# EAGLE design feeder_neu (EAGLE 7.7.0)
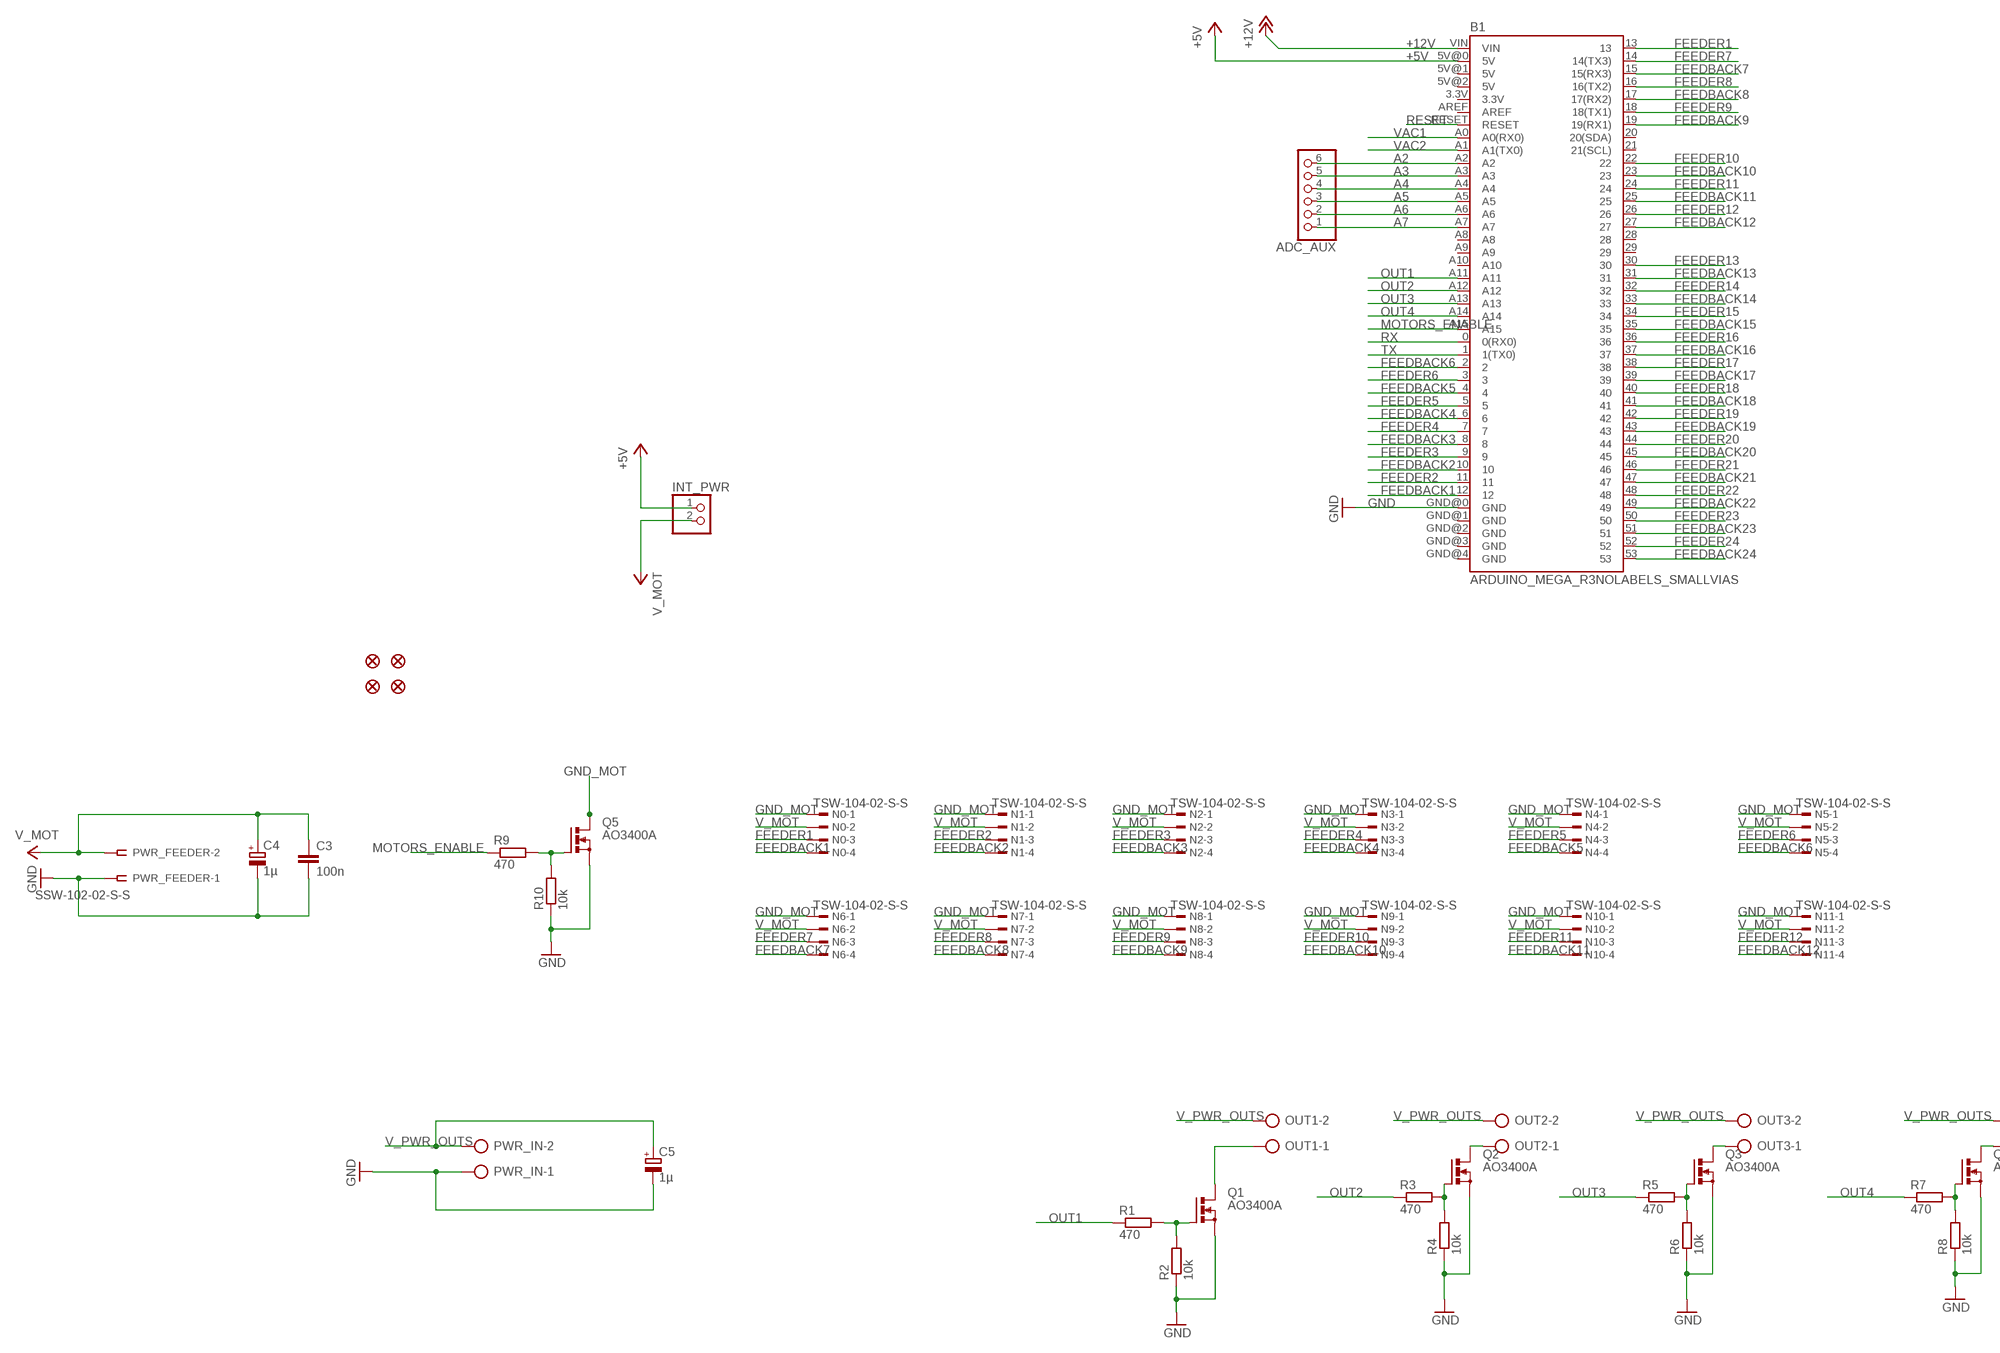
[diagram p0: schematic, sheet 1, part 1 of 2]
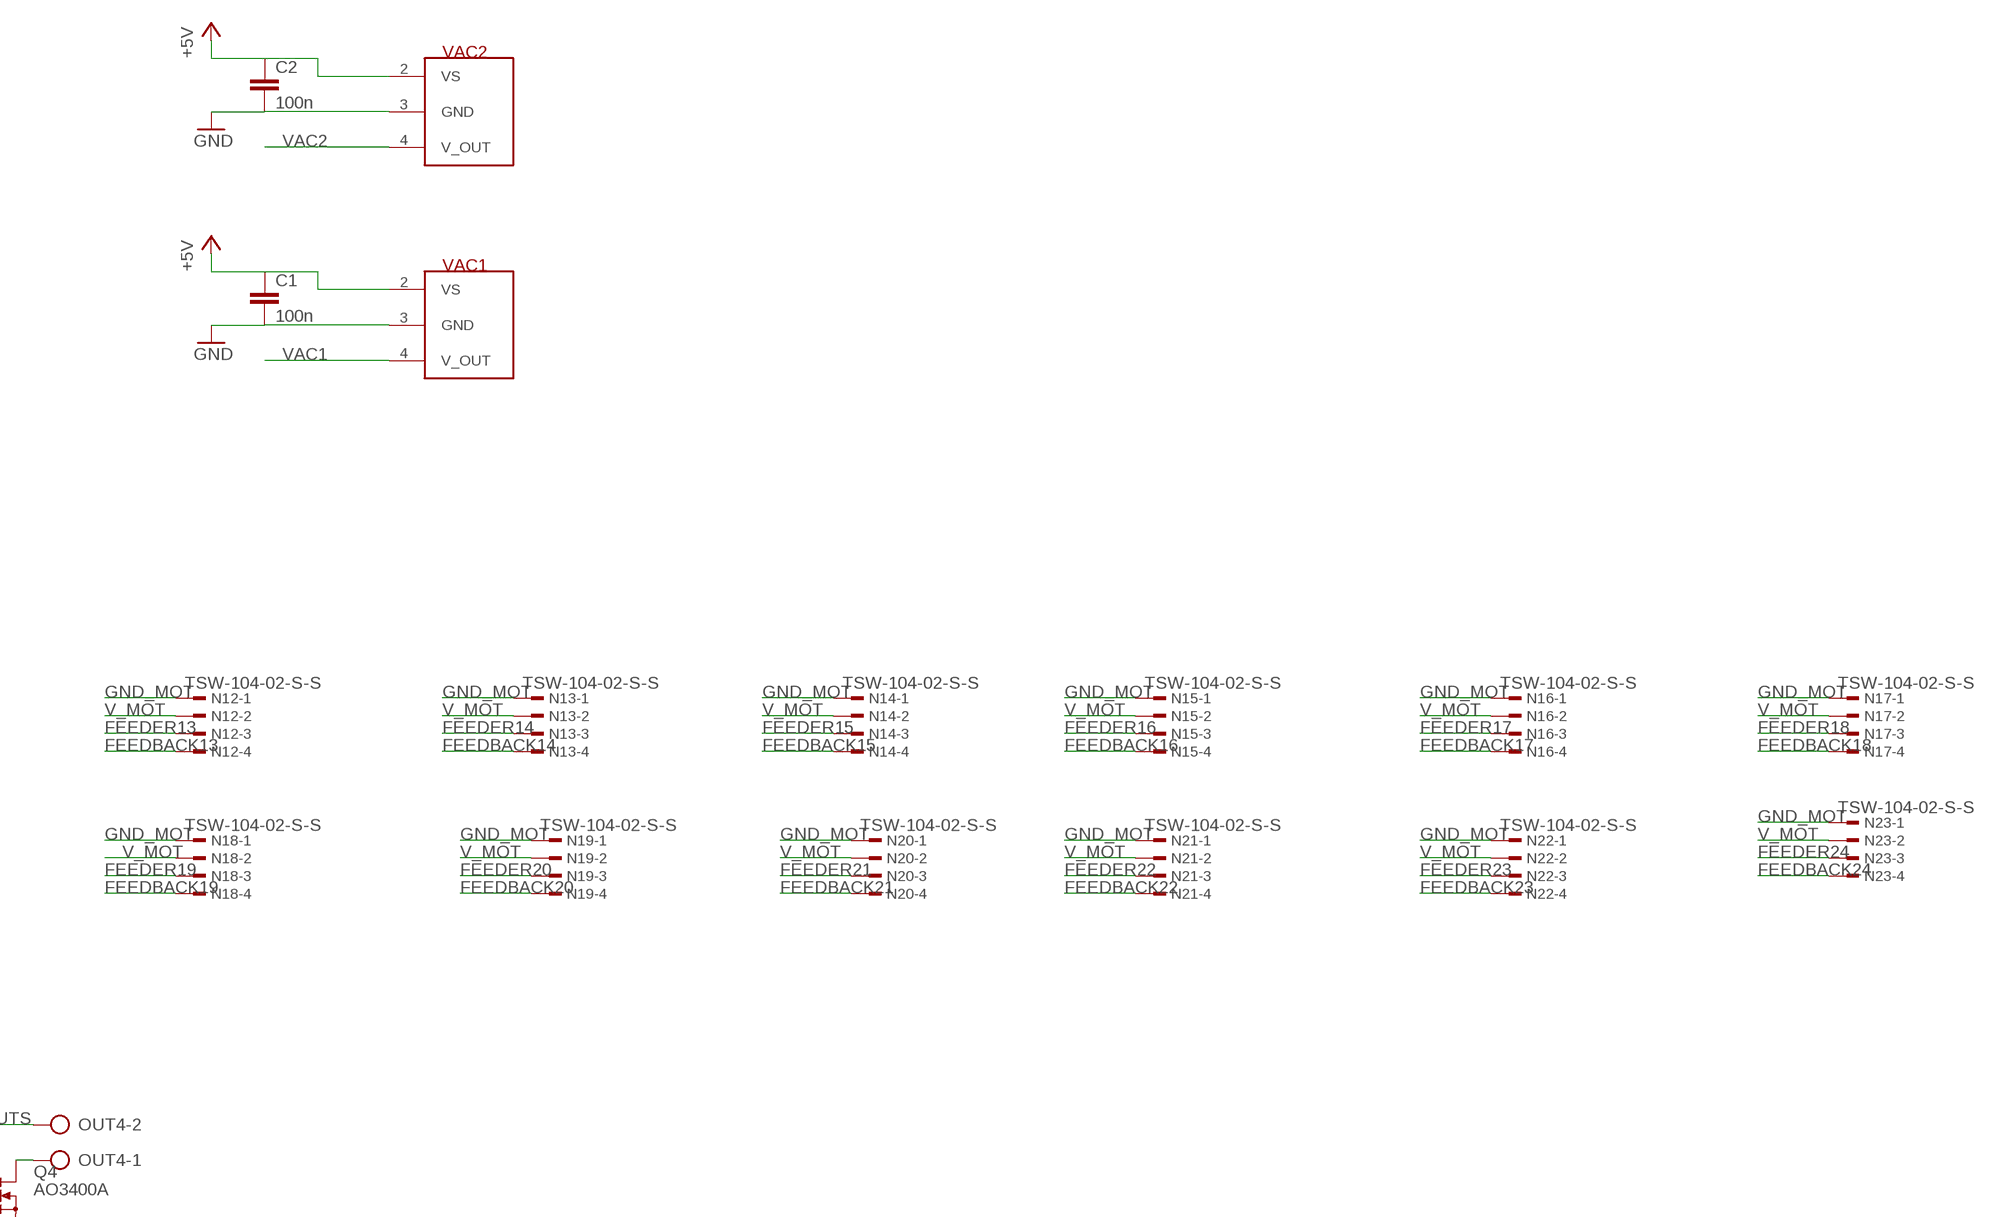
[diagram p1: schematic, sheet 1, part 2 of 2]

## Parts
ADC_AUX  PINHD-1X6  [1X06]
B1  ARDUINO_MEGA_R3NOLABELS_SMALLVIAS  [ARDUINO_MEGA_NOLABELS_SMALLVIAS]
C1  100n  C-EUC0603K  [C0603K]
C2  100n  C-EUC0603K  [C0603K]
C3  100n  C-EUC0603K  [C0603K]
C4  1µ  CPOL-EUE2.5-5  [E2,5-5]
C5  1µ  CPOL-EUE2.5-5  [E2,5-5]
FD1  FIDUCIAL1X2  [FIDUCIAL-1X2]
FD2  FIDUCIAL1X2  [FIDUCIAL-1X2]
FD3  FIDUCIAL1X2  [FIDUCIAL-1X2]
FD4  FIDUCIAL1X2  [FIDUCIAL-1X2]
INT_PWR  PINHD-1X2  [1X02]
N0  TSW-104-02-S-S  [TSW-104-02-S-S]
N1  TSW-104-02-S-S  [TSW-104-02-S-S]
N2  TSW-104-02-S-S  [TSW-104-02-S-S]
N3  TSW-104-02-S-S  [TSW-104-02-S-S]
N4  TSW-104-02-S-S  [TSW-104-02-S-S]
N5  TSW-104-02-S-S  [TSW-104-02-S-S]
N6  TSW-104-02-S-S  [TSW-104-02-S-S]
N7  TSW-104-02-S-S  [TSW-104-02-S-S]
N8  TSW-104-02-S-S  [TSW-104-02-S-S]
N9  TSW-104-02-S-S  [TSW-104-02-S-S]
N10  TSW-104-02-S-S  [TSW-104-02-S-S]
N11  TSW-104-02-S-S  [TSW-104-02-S-S]
N12  TSW-104-02-S-S  [TSW-104-02-S-S]
N13  TSW-104-02-S-S  [TSW-104-02-S-S]
N14  TSW-104-02-S-S  [TSW-104-02-S-S]
N15  TSW-104-02-S-S  [TSW-104-02-S-S]
N16  TSW-104-02-S-S  [TSW-104-02-S-S]
N17  TSW-104-02-S-S  [TSW-104-02-S-S]
N18  TSW-104-02-S-S  [TSW-104-02-S-S]
N19  TSW-104-02-S-S  [TSW-104-02-S-S]
N20  TSW-104-02-S-S  [TSW-104-02-S-S]
N21  TSW-104-02-S-S  [TSW-104-02-S-S]
N22  TSW-104-02-S-S  [TSW-104-02-S-S]
N23  TSW-104-02-S-S  [TSW-104-02-S-S]
OUT1  AK500/2  [AK500/2]
OUT2  AK500/2  [AK500/2]
OUT3  AK500/2  [AK500/2]
OUT4  AK500/2  [AK500/2]
PWR_FEEDER  SSW-102-02-S-S  [SSW-102-02-S-S]
PWR_IN  AK500/2  [AK500/2]
Q1  AO3400A  [SOT23]
Q2  AO3400A  [SOT23]
Q3  AO3400A  [SOT23]
Q4  AO3400A  [SOT23]
Q5  AO3400A  [SOT23]
R1  470  R-EU_R0805  [R0805]
R2  10k  R-EU_R0805  [R0805]
R3  470  R-EU_R0805  [R0805]
R4  10k  R-EU_R0805  [R0805]
R5  470  R-EU_R0805  [R0805]
R6  10k  R-EU_R0805  [R0805]
R7  470  R-EU_R0805  [R0805]
R8  10k  R-EU_R0805  [R0805]
R9  470  R-EU_R0805  [R0805]
R10  10k  R-EU_R0805  [R0805]
VAC1  MPXV6115VC6U  [MPXV6115VC6U]
VAC2  MPXV6115VC6U  [MPXV6115VC6U]

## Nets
+5V: B1.5V@0(5V) C1.1 C2.1 INT_PWR.1 VAC1.2(VS) VAC2.2(VS)
+12V: B1.VIN
A2: ADC_AUX.6 B1.A2
A3: ADC_AUX.5 B1.A3
A4: ADC_AUX.4 B1.A4
A5: ADC_AUX.3 B1.A5
A6: ADC_AUX.2 B1.A6
A7: ADC_AUX.1 B1.A7
FEEDBACK1: B1.12 N0.4
FEEDBACK2: B1.10 N1.4
FEEDBACK3: B1.8 N2.4
FEEDBACK4: B1.6 N3.4
FEEDBACK5: B1.4 N4.4
FEEDBACK6: B1.2 N5.4
FEEDBACK7: B1.15(15(RX3)) N6.4
FEEDBACK8: B1.17(17(RX2)) N7.4
FEEDBACK9: B1.19(19(RX1)) N8.4
FEEDBACK10: B1.23 N9.4
FEEDBACK11: B1.25 N10.4
FEEDBACK12: B1.27 N11.4
FEEDBACK13: B1.31 N12.4
FEEDBACK14: B1.33 N13.4
FEEDBACK15: B1.35 N14.4
FEEDBACK16: B1.37 N15.4
FEEDBACK17: B1.39 N16.4
FEEDBACK18: B1.41 N17.4
FEEDBACK19: B1.43 N18.4
FEEDBACK20: B1.45 N19.4
FEEDBACK21: B1.47 N20.4
FEEDBACK22: B1.49 N21.4
FEEDBACK23: B1.51 N22.4
FEEDBACK24: B1.53 N23.4
FEEDER1: B1.13 N0.3
FEEDER2: B1.11 N1.3
FEEDER3: B1.9 N2.3
FEEDER4: B1.7 N3.3
FEEDER5: B1.5 N4.3
FEEDER6: B1.3 N5.3
FEEDER7: B1.14(14(TX3)) N6.3
FEEDER8: B1.16(16(TX2)) N7.3
FEEDER9: B1.18(18(TX1)) N8.3
FEEDER10: B1.22 N9.3
FEEDER11: B1.24 N10.3
FEEDER12: B1.26 N11.3
FEEDER13: B1.30 N12.3
FEEDER14: B1.32 N13.3
FEEDER15: B1.34 N14.3
FEEDER16: B1.36 N15.3
FEEDER17: B1.38 N16.3
FEEDER18: B1.40 N17.3
FEEDER19: B1.42 N18.3
FEEDER20: B1.44 N19.3
FEEDER21: B1.46 N20.3
FEEDER22: B1.48 N21.3
FEEDER23: B1.50 N22.3
FEEDER24: B1.52 N23.3
GND: B1.GND@0(GND) C1.2 C2.2 C3.2 C4.- C5.- PWR_FEEDER.1 PWR_IN.1 Q1.2(S) Q2.2(S) Q3.2(S) Q4.2(S) Q5.2(S) R2.1 R4.1 R6.1 R8.1 R10.1 VAC1.3(GND) VAC2.3(GND)
GND_MOT: N0.1 N1.1 N2.1 N3.1 N4.1 N5.1 N6.1 N7.1 N8.1 N9.1 N10.1 N11.1 N12.1 N13.1 N14.1 N15.1 N16.1 N17.1 N18.1 N19.1 N20.1 N21.1 N22.1 N23.1 Q5.3(D)
MOTORS_ENABLE: B1.A15 R9.1
N$1: Q1.1(G) R1.2 R2.2
N$2: OUT4.1 Q4.3(D)
N$3: Q5.1(G) R9.2 R10.2
N$4: OUT1.1 Q1.3(D)
N$7: OUT2.1 Q2.3(D)
N$8: OUT3.1 Q3.3(D)
N$10: Q4.1(G) R7.2 R8.2
N$13: Q3.1(G) R5.2 R6.2
N$14: Q2.1(G) R3.2 R4.2
OUT1: B1.A11 R1.1
OUT2: B1.A12 R3.1
OUT3: B1.A13 R5.1
OUT4: B1.A14 R7.1
RESET: B1.RESET
RX: B1.0(0(RX0))
TX: B1.1(1(TX0))
V_MOT: C3.1 C4.+ INT_PWR.2 N0.2 N1.2 N2.2 N3.2 N4.2 N5.2 N6.2 N7.2 N8.2 N9.2 N10.2 N11.2 N12.2 N13.2 N14.2 N15.2 N16.2 N17.2 N18.2 N19.2 N20.2 N21.2 N22.2 N23.2 PWR_FEEDER.2
V_PWR_OUTS: C5.+ OUT1.2 OUT2.2 OUT3.2 OUT4.2 PWR_IN.2
VAC1: B1.A0(A0(RX0)) VAC1.4(V_OUT)
VAC2: B1.A1(A1(TX0)) VAC2.4(V_OUT)
Unconnected: B1.3.3V B1.5V@1(5V) B1.5V@2(5V) B1.20(20(SDA)) B1.21(21(SCL)) B1.28 B1.29 B1.A8 B1.A9 B1.A10 B1.AREF B1.GND@1(GND) B1.GND@2(GND) B1.GND@3(GND) B1.GND@4(GND)

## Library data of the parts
ADC_AUX = pinhead:PINHD-1X6: PIN HEADER
B1 = SparkFun-Boards:ARDUINO_MEGA_R3: Arduino Mega R3 ATmega2560 R3 compatible footprint. SparkFun Products: Arduino Mega 2560 R3
C1-C3 = resistor:C-EU: CAPACITOR, European symbol
C4 C5 = rcl:CPOL-EU: POLARIZED CAPACITOR, European symbol
FD1-FD4 = SparkFun-Aesthetics:FIDUCIAL: Fiducial Alignment Points
INT_PWR = pinhead:PINHD-1X2: PIN HEADER
N0 N1-N23 = con-samtec:TSW-104-02-S-S: THROUGH-HOLE .025" SQ POST HEADER Source: Samtec TSW.pdf; OC_FARNELL: unknown; OC_NEWARK: unknown
OUT1-OUT4 PWR_IN = con-ptr500:AK500/2: CONNECTOR; OC_FARNELL: unknown; OC_NEWARK: unknown
PWR_FEEDER = con-samtec:SSW-102-02-S-S: THROUGH-HOLE .025" SQ POST SOCKET; MPN: SSW-102-02-S-S; OC_FARNELL: unknown; OC_NEWARK: 11P9351
Q1-Q5 = mosfets:AO3400A: N-CHANNEL MOS FET
R1-R10 = resistor:R-EU_: RESISTOR, European symbol
VAC1 VAC2 = sensors:MPXV6115VC6U

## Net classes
0 default: clearance 0.205 mm
2 ledpower: width 0.102 mm, clearance 0.205 mm to class 0, clearance 0.205 mm to class 1, clearance 0.205 mm

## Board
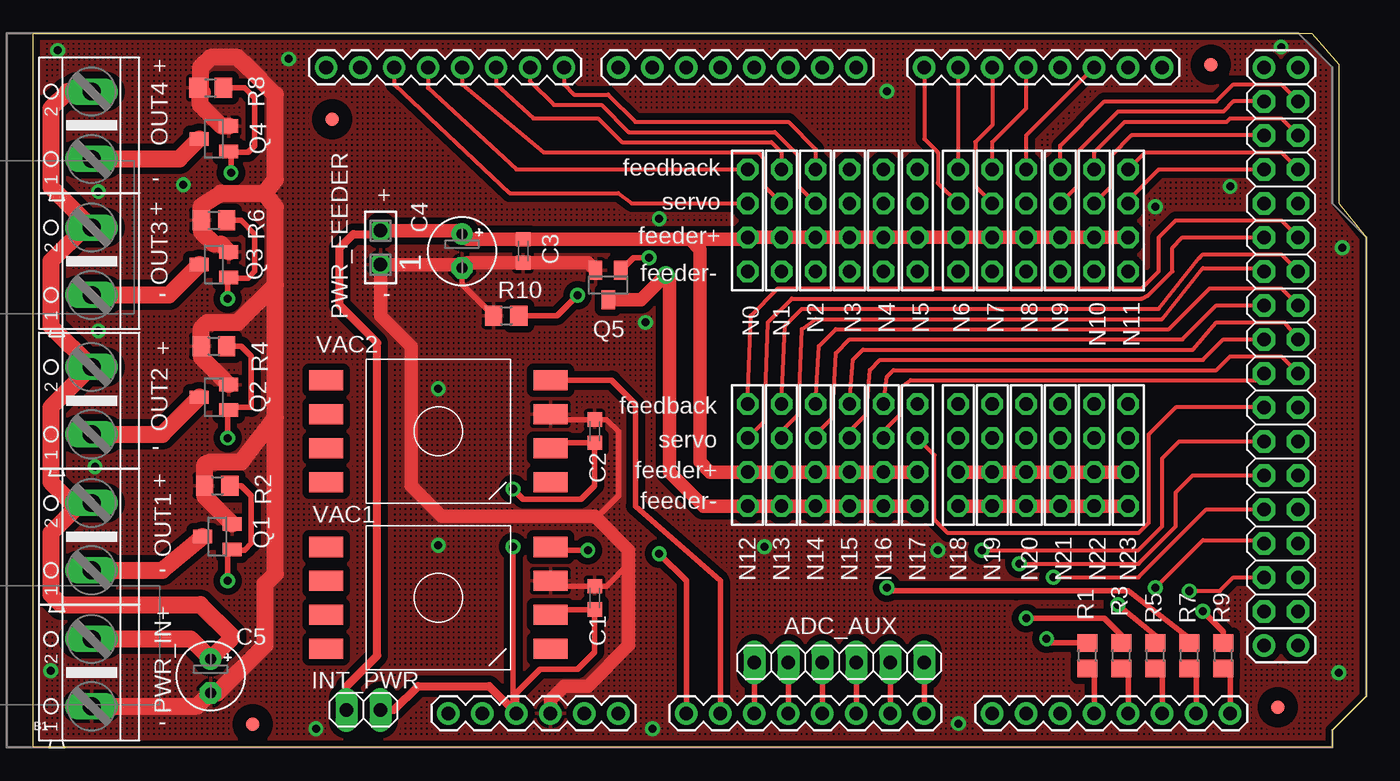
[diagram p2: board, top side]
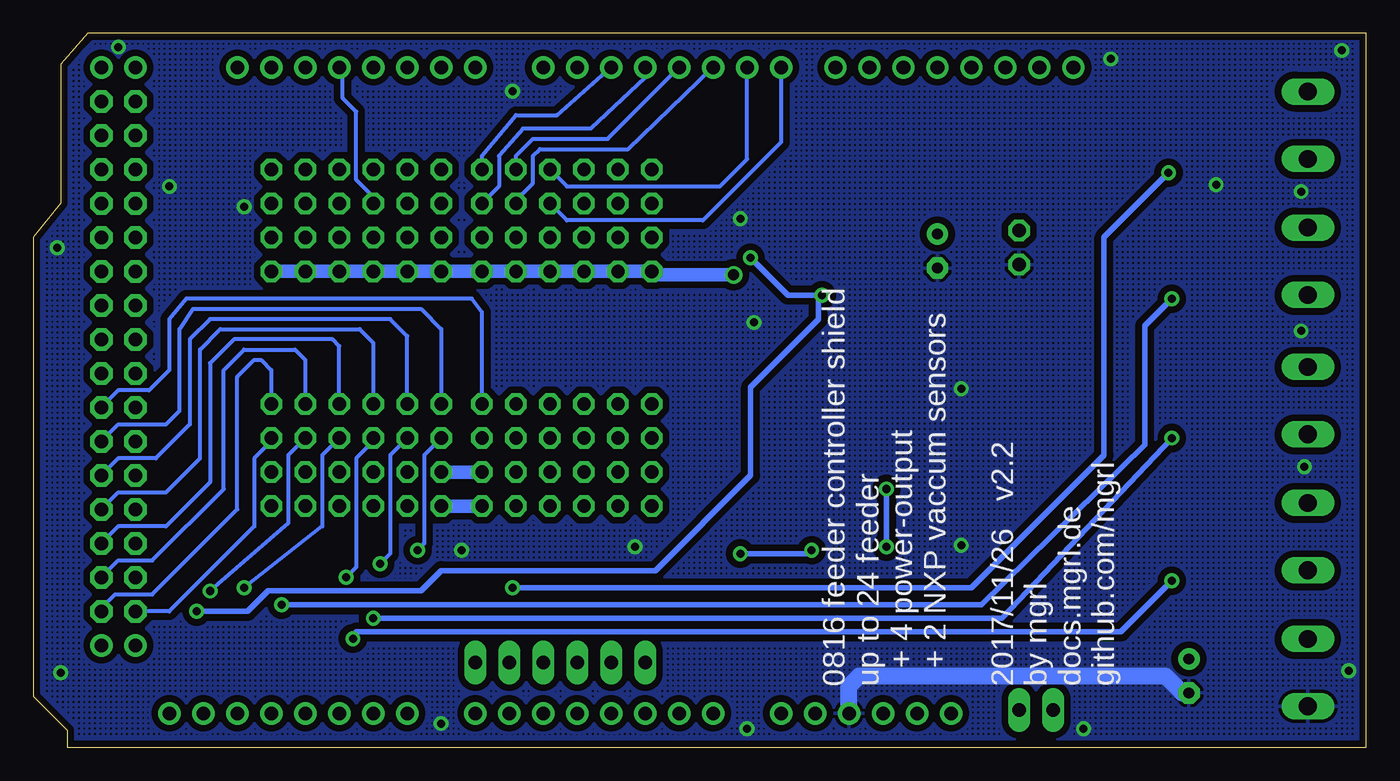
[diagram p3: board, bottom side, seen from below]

Size 99.6 x 53.34 mm. Coordinates in mm from the lower left corner, seen from the top.
Outline: 0,0 0,53.34 95.54,53.34 97.57,51.05 97.57,40.64 99.6,38.1 99.6,3.81 97.06,1.27 97.06,0 0,0
Copper layers (1*16): Top 0.035mm / dielectric 1.5mm / Bottom 0.035mm
Design rules "SparkFun": minimum track width 8mil, minimum drill 20mil, track to track 8mil, track to pad 8mil, pad to pad 8mil, via to via 8mil, smd to smd 8mil, copper to edge 8mil, drill to drill 8mil, minimum pad ring 12mil, minimum via ring 10mil, stop-mask expansion 4mil, vias tented up to drill 20mil, thermal gap 10mil

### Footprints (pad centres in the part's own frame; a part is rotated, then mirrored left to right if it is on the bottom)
1X06 = drill 1.016 long: 1 -6.35,0; 2 -3.81,0; 3 -1.27,0; 4 1.27,0; 5 3.81,0; 6 6.35,0
ARDUINO_MEGA_NOLABELS_SMALLVIAS = drill 1.016 pad 1.676: 0 13.97,24.13; 1 11.43,24.13; 2 8.89,24.13; 3 6.35,24.13; 3.3V -13.97,-24.13; 4 3.81,24.13; 5 1.27,24.13; 5V@0 -11.43,-24.13; 5V@1 44.45,24.13; 5V@2 46.99,24.13; 6 -1.27,24.13; 7 -3.81,24.13; 8 -7.874,24.13; 9 -10.414,24.13; 10 -12.954,24.13; 11 -15.494,24.13; 12 -18.034,24.13; 13 -20.574,24.13; 14 19.05,24.13; 15 21.59,24.13; 16 24.13,24.13; 17 26.67,24.13; 18 29.21,24.13; 19 31.75,24.13; 20 34.29,24.13; 21 36.83,24.13; A0 1.27,-24.13; A1 3.81,-24.13; A2 6.35,-24.13; A3 8.89,-24.13; A4 11.43,-24.13; A5 13.97,-24.13; A6 16.51,-24.13; A7 19.05,-24.13; A8 24.13,-24.13; A9 26.67,-24.13; A10 29.21,-24.13; A11 31.75,-24.13; A12 34.29,-24.13; A13 36.83,-24.13; A14 39.37,-24.13; A15 41.91,-24.13; AREF -25.654,24.13; GND@0 -8.89,-24.13; GND@1 -6.35,-24.13; GND@2 44.45,-19.05; GND@3 46.99,-19.05; GND@4 -23.114,24.13; RESET -16.51,-24.13; VIN -3.81,-24.13 | drill 1.016 pad 1.676 octagon: 22 44.45,21.59; 23 46.99,21.59; 24 44.45,19.05; 25 46.99,19.05; 26 44.45,16.51; 27 46.99,16.51; 28 44.45,13.97; 29 46.99,13.97; 30 44.45,11.43; 31 46.99,11.43; 32 44.45,8.89; 33 46.99,8.89; 34 44.45,6.35; 35 46.99,6.35; 36 44.45,3.81; 37 46.99,3.81; 38 44.45,1.27; 39 46.99,1.27; 40 44.45,-1.27; 41 46.99,-1.27; 42 44.45,-3.81; 43 46.99,-3.81; 44 44.45,-6.35; 45 46.99,-6.35; 46 44.45,-8.89; 47 46.99,-8.89; 48 44.45,-11.43; 49 46.99,-11.43; 50 44.45,-13.97; 51 46.99,-13.97; 52 44.45,-16.51; 53 46.99,-16.51
C0603K = smd 1.05 x 1.08: 1 -0.875,0; 2 0.875,0
E2,5-5 = drill 0.813 pad 1.6: + -1.27,0 | drill 0.813 pad 1.6 octagon: - 1.27,0
FIDUCIAL-1X2 = smd 1 x 1: 1 0,0
1X02 = drill 1.016 long: 1 -1.27,0; 2 1.27,0
TSW-104-02-S-S = drill 1 pad 1.5 octagon: 1 3.81,0; 2 1.27,0; 3 -1.27,0; 4 -3.81,0
AK500/2 = drill 1.321 long: 1 -2.515,0; 2 2.515,0
SSW-102-02-S-S = drill 1 pad 1.5 octagon: 1 -1.27,0; 2 1.27,0
SOT23 = smd 1 x 1.4: 1 -0.95,-1.1; 2 0.95,-1.1; 3 0,1.1
R0805 = smd 1.3 x 1.5: 1 -0.95,0; 2 0.95,0
MPXV6115VC6U = smd 2.54 x 1.524: 1 8.382,-3.81; 2 8.382,-1.27; 3 8.382,1.27; 4 8.382,3.81; 5 -8.382,-3.81; 6 -8.382,-1.27; 7 -8.382,1.27; 8 -8.382,3.81

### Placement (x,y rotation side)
ADC_AUX  60.23,6.35 180 top
B1  47.53,26.67 0 top
C1  41.94,11.18 90 top
C2  41.94,23.62 90 top
C3  36.61,37.08 270 top
C4  32.04,37.08 270 top
C5  13.24,5.33 270 top
FD1  16.38,1.73 0 top
FD2  22.32,46.94 0 top
FD3  93,3 0 top
FD4  88,51 0 top
INT_PWR  24.67,2.79 180 top
N0  53.37,39.37 270 top
N1  55.91,39.37 270 top
N2  58.45,39.37 270 top
N3  60.99,39.37 270 top
N4  63.53,39.37 270 top
N5  66.07,39.37 270 top
N6  69.12,39.37 270 top
N7  71.66,39.37 270 top
N8  74.2,39.37 270 top
N9  76.74,39.37 270 top
N10  79.28,39.37 270 top
N11  81.82,39.37 270 top
N12  53.37,21.84 270 top
N13  55.91,21.84 270 top
N14  58.45,21.84 270 top
N15  60.99,21.84 270 top
N16  63.53,21.84 270 top
N17  66.07,21.84 270 top
N18  69.12,21.84 270 top
N19  71.66,21.84 270 top
N20  74.2,21.84 270 top
N21  76.74,21.84 270 top
N22  79.28,21.84 270 top
N23  81.82,21.84 270 top
OUT1  4.35,15.75 90 top
OUT2  4.35,25.91 90 top
OUT3  4.35,36.32 90 top
OUT4  4.35,46.48 90 top
PWR_FEEDER  25.94,37.34 90 top
PWR_IN  4.35,5.59 90 top
Q1  13.75,15.75 90 top
Q2  13.49,26.16 90 top
Q3  13.49,36.07 90 top
Q4  13.49,45.47 90 top
Q5  42.96,34.54 180 top
R1  78.77,6.86 90 top
R2  13.75,19.56 0 top
R3  81.31,6.86 90 top
R4  13.49,29.97 0 top
R5  83.85,6.86 90 top
R6  13.49,39.37 0 top
R7  86.39,6.86 90 top
R8  13.24,49.28 0 top
R9  88.93,6.86 90 top
R10  35.34,32.26 0 top
VAC1  30.26,11.18 0 top
VAC2  30.26,23.62 0 top

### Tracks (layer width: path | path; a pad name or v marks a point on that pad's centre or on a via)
+5V  (via drill 0.6)
  Top 0.406: VAC1.2 39.03,10.3 C1.1 41.94,7.11 40.67,5.84 37.88,5.84 36.1,4.06 B1.5V@0 35.85,2.79 v35.85,14.99 | v35.85,19.3 36.61,18.54 40.93,18.54 41.94,19.56 C2.1 39.03,22.75 VAC2.2
  Top 0.61: INT_PWR.1 26.96,2.79 28.73,4.57 34.07,4.57 B1.5V@0
  Bottom 0.406: v35.85,19.3 v35.85,14.99
A2
  Top 0.406: B1.A2 ADC_AUX.6
A3
  Top 0.406: B1.A3 ADC_AUX.5
A4
  Top 0.406: B1.A4 ADC_AUX.4
A5
  Top 0.406: B1.A5 ADC_AUX.3
A6
  Top 0.406: B1.A6 ADC_AUX.2
A7
  Top 0.406: B1.A7 ADC_AUX.1
FEEDBACK1
  Top 0.305: B1.12 29.5,49.28 36.1,43.18 37.12,43.18 50.32,43.18 N0.4
FEEDBACK2
  Top 0.305: B1.10 34.58,49.53 37.37,46.99 42.2,46.99 43.97,45.21 55.15,45.21 55.91,44.45 N1.4
FEEDBACK3
  Top 0.305: B1.8 39.66,49.53 40.42,48.77 42.96,48.77 44.99,46.74 56.42,46.74 58.45,44.7 N2.4
FEEDBACK4
  Bottom 0.305: N3.4 59.72,41.91 48.29,41.91 46.26,43.94 B1.6
FEEDBACK5
  Bottom 0.305: N4.4 63.53,44.2 62.26,45.47 56.67,45.47 B1.4
FEEDBACK6
  Bottom 0.305: N5.4 66.07,44.2 63.53,47.24 60.48,47.24 B1.2
FEEDBACK7
  Top 0.305: N6.4 B1.15
FEEDBACK8
  Top 0.305: N7.4 71.66,45.21 74.2,47.75 B1.17
FEEDBACK9
  Top 0.305: N8.4 74.2,45.72 B1.19
FEEDBACK10
  Top 0.305: N9.4 76.74,44.96 80.04,48.26 88.42,48.26 89.69,49.53 93.25,49.53 B1.23
FEEDBACK11
  Top 0.305: N10.4 79.28,44.45 81.57,46.74 89.19,46.74 89.44,46.99 93.25,46.99 B1.25
FEEDBACK12
  Top 0.305: N11.4 83.09,44.45 92.23,44.45 93.25,44.45 B1.27
FEEDBACK13
  Top 0.305: N12.4 53.63,32.26 55.66,34.29 82.84,34.29 84.11,35.56 84.11,38.1 85.38,39.37 93.25,39.37 B1.31
FEEDBACK14
  Top 0.305: N13.4 56.17,31.5 57.44,32.77 84.11,32.77 87.15,36.58 87.41,36.83 93.25,36.83 B1.33
FEEDBACK15
  Top 0.305: N14.4 58.71,29.97 59.98,31.24 84.87,31.24 87.92,34.29 93.25,34.29 B1.35
FEEDBACK16
  Top 0.305: N15.4 61.25,28.96 62.01,29.72 86.65,29.72 88.42,31.75 93.5,31.75 B1.37
FEEDBACK17
  Top 0.305: N16.4 63.79,27.69 64.29,28.19 88.42,28.19 89.44,29.21 93.25,29.21 B1.39
FEEDBACK18
  Bottom 0.305: N17.4 66.07,32.51 66.83,33.53 88.17,33.53 89.44,32 89.44,28.19 90.96,26.67 93.25,26.67 B1.41
FEEDBACK19
  Bottom 0.305: B1.43 93.25,24.13 89.69,24.13 88.68,25.15 88.68,31.24 87.66,32.77 70.64,32.77 69.12,31.24 N18.4
FEEDBACK20
  Bottom 0.305: N19.4 71.66,30.73 72.93,32 86.39,32 87.92,30.48 87.92,24.13 90.46,21.59 93.25,21.59 B1.45
FEEDBACK21
  Bottom 0.305: B1.47 93.25,19.05 89.69,19.05 87.15,21.59 87.15,29.72 85.63,31.24 75.22,31.24 74.2,30.23 N20.4
FEEDBACK22
  Bottom 0.305: N21.4 76.74,29.97 77.25,30.48 84.61,30.48 86.39,28.7 86.39,19.81 89.69,16.51 93.25,16.51 B1.49
FEEDBACK23
  Bottom 0.305: B1.51 93.25,13.97 90.71,13.97 85.38,19.3 85.38,28.19 83.85,29.72 80.04,29.72 79.28,28.96 N22.4
FEEDBACK24
  Bottom 0.305: B1.53 94.52,10.41 93.5,11.43 90.71,11.43 84.36,17.78 84.36,27.69 83.09,28.96 82.58,28.96 81.82,28.19 N23.4
FEEDER1
  Top 0.305: B1.13 26.96,49.53 35.59,41.4 43.72,41.4 44.74,40.64 N0.3
FEEDER2
  Top 0.305: B1.11 32.04,49.53 38.13,44.45 49.05,44.45 52.36,44.45 54.13,44.45 54.64,43.94 54.64,41.91 N1.3
FEEDER3
  Top 0.305: B1.9 37.12,49.78 38.89,48.01 42.45,48.01 44.48,45.97 55.4,45.97 57.18,44.2 57.18,41.91 N2.3
FEEDER4
  Bottom 0.305: B1.7 43.72,45.21 49.56,39.37 59.72,39.37 N3.3
FEEDER5
  Bottom 0.305: N4.3 63.53,40.89 62.26,42.16 62.26,44.2 61.75,44.7 55.15,44.7 B1.5
FEEDER6
  Bottom 0.305: B1.3 53.88,50.04 57.94,46.23 63.02,46.23 64.8,44.2 64.8,41.91 N5.3
FEEDER7
  Top 0.305: B1.14 66.58,45.47 67.6,44.45 67.6,42.16 N6.3
FEEDER8
  Top 0.305: B1.16 71.66,46.48 70.39,45.21 70.39,41.91 N7.3
FEEDER9
  Bottom 0.305: N8.3 74.2,41.15 75.47,42.42 75.47,47.5 76.49,48.51 76.49,50.55 B1.18
FEEDER10
  Top 0.305: B1.22 89.69,48.26 88.93,47.5 81.06,47.5 78.01,44.45 78.01,41.91 N9.3
FEEDER11
  Top 0.305: B1.24 82.07,45.72 80.55,44.2 80.55,41.91 N10.3
FEEDER12
  Top 0.305: N11.3 81.82,40.89 84.11,43.18 B1.26
FEEDER13
  Top 0.305: N12.3 54.64,24.38 54.9,31.75 56.67,33.53 82.84,33.53 83.34,33.78 85.12,35.56 85.12,37.34 85.88,38.1 B1.30
FEEDER14
  Top 0.305: N13.3 55.91,23.62 57.18,24.89 57.44,31.24 58.45,32 84.36,32 87.41,35.81 91.73,35.81 B1.32
FEEDER15
  Top 0.305: N14.3 58.45,23.37 59.72,24.64 59.98,29.46 60.99,30.48 85.88,30.48 88.42,33.02 B1.34
FEEDER16
  Top 0.305: N15.3 60.99,23.62 62.26,24.89 62.52,28.19 63.28,28.96 87.41,28.96 88.93,30.48 B1.36
FEEDER17
  Top 0.305: N16.3 63.53,23.62 64.8,24.89 64.8,26.92 65.56,27.43 91.47,27.43 91.73,27.69 B1.38
FEEDER18
  Top 0.305: B1.40 85.38,25.4 83.34,23.37 83.34,16.76 82.58,16 68.36,16 67.34,17.02 67.34,21.84 N17.3
FEEDER19  (via drill 0.6)
  Top 0.305: v70.9,14.73 82.58,14.73 84.36,16.51 84.36,21.59 85.63,22.86 B1.42
  Bottom 0.305: N18.3 70.39,21.84 70.39,15.24 v70.9,14.73
FEEDER20  (via drill 0.6)
  Top 0.305: v73.69,13.72 82.58,13.72 85.38,16.51 85.38,19.05 86.65,20.32 B1.44
  Bottom 0.305: N19.3 72.93,21.84 72.93,14.48 v73.69,13.72
FEEDER21  (via drill 0.6)
  Top 0.305: v76.23,12.7 82.58,12.7 87.66,17.78 B1.46
  Bottom 0.305: N20.3 74.2,22.86 75.47,21.59 75.47,13.46 v76.23,12.7
FEEDER22  (via drill 0.6)
  Top 0.305: v83.85,11.94 87.41,15.49 91.73,15.49 B1.48
  Bottom 0.305: N21.3 78.01,21.84 78.01,16.51 v83.85,11.94
FEEDER23  (via drill 0.6)
  Top 0.305: v86.39,11.68 88.68,11.68 89.69,12.7 B1.50
  Bottom 0.305: N22.3 80.55,21.84 80.55,16.76 v86.39,11.68
FEEDER24
  Bottom 0.305: N23.3 81.82,22.86 83.09,21.59 83.09,16.51 89.44,10.16 B1.52
GND  (via drill 0.6)
  Top 0.406: 12.73,48.83 12.64,48.93 R8.1 | R6.1 12.54,38.54 | 13.49,37.59 14.02,37.59 | R2.1 12.8,18.75 | R4.1 12.54,29.16 | VAC1.3 39.03,12.05 C1.2 42.82,12.05 44.48,13.72 | VAC2.3 39.03,24.5 C2.2 42.84,24.5 43.72,23.62 43.72,18.8 42.07,17.14 | C4.- 32.04,34.61 R10.1
  Top 1.016: Q5.2 41.44,36.21 C3.2 32.43,36.21 C4.- 31.78,36.07 PWR_FEEDER.1 25.94,32.26 28.23,29.97 28.23,19.56 30.51,17.27 41.94,17.27 42.07,17.14 44.48,14.73 44.48,13.72 44.48,7.62 41.43,4.57 39.66,4.57 38.64,3.56 B1.GND@0
  Top 1.27: Q4.2 14.07,46.42 12.48,48.01 12.48,48.77 | 12.54,38.54 13.49,37.59 | 14.02,37.59 Q3.2 | 12.8,18.75 Q1.2 | 12.54,29.16 Q2.2 | PWR_IN.1 12.25,3.07 C5.- 13.75,4.06 17.3,7.62 17.3,12.19 18.07,12.95 18.07,24.64 | 12.48,48.77 12.64,48.93 | R6.1 12.54,40.45 14,41.4 17.3,41.4 | 17.3,41.4 18.07,42.42 18.07,48.77 16.03,50.8 15.27,51.56 13.24,51.56 12.48,50.8 12.48,48.77 | R4.1 12.54,31.31 12.99,31.75 15.27,31.75 18.07,34.54 | 18.07,34.54 18.07,40.39 17.3,41.4 | R2.1 12.8,21.15 13.24,21.34 15.53,21.34 18.07,24.64 | 18.07,24.64 18.07,34.54
  Bottom 1.27: B1.GND@0 38.64,4.57 37.88,5.33 15.02,5.33 13.75,4.06 C5.-
  other vias: 1.81,52.07 63.79,49.02 89.44,41.91 83.85,40.39 93.25,52.32 97.82,37.34 97.57,5.59 69.12,1.78 54.64,14.99 45.75,31.75 46.77,39.5 19.08,51.44 11.21,42.04 4.86,31.11 4.86,41.53 4.6,20.95 1.3,5.71 21.11,1.4 46.26,1.4 30.26,26.8 30.26,15.11 67.6,14.73
  pour Top (isolate 0.5, hatched): -0.22,53.34 0.03,0 97.06,0 97.06,1.27 99.6,3.81 99.6,38.1 97.06,40.64 97.06,50.8 94.52,53.34
  pour Bottom (isolate 0.5, hatched): -0.22,53.34 94.52,53.34 97.06,50.8 97.06,40.64 99.6,38.1 99.6,3.81 97.06,1.27 97.06,0 0.03,0
GND_MOT  (via drill 0.8)
  Top 1.016: Q5.3 45.41,33.44 v47.28,35.31 47.53,35.05 47.53,20.57 50.07,18.03 N12.1 N13.1 N14.1 N15.1 N16.1 N17.1 | N18.1 N19.1 N20.1 N21.1 N22.1 N23.1
  Bottom 1.016: v47.28,35.31 53.12,35.31 N0.1 N1.1 N2.1 N3.1 N4.1 N5.1 N6.1 N7.1 N8.1 N9.1 N10.1 N11.1 | N17.1 N18.1
MOTORS_ENABLE
  Top 0.406: B1.A15 89.44,5.4 R9.1
N$1  (via drill 0.6)
  Top 0.406: R1.2 76.04,7.81 v75.72,8.13 | v14.51,12.45 14.51,14.63 Q1.1 14.41,14.73 15.78,14.73 16.29,15.24 16.29,18.8 15.53,19.56 R2.2
  Bottom 0.406: v75.72,8.13 75.72,8.38 75.47,8.64 18.32,8.64 v14.51,12.45
N$2
  Top 1.27: OUT4.1 10.89,43.97 Q4.3
N$3  (via drill 0.6)
  Top 0.406: R10.2 39.15,32.26 v40.67,33.78 | v46.01,36.58 44.84,36.58 Q5.1 | R9.2 88.93,8.64 v87.41,10.16
  Bottom 0.406: v46.01,36.58 43.21,33.78 v40.67,33.78 40.93,33.53 40.93,32 46.01,26.92 46.01,20.32 53.12,13.21 69.12,13.21 70.64,11.68 82.07,11.68 83.6,10.16 v87.41,10.16
N$4
  Top 1.27: OUT1.1 9.62,13.23 Q1.3
N$7
  Top 1.27: OUT2.1 9.62,23.39 Q2.3
N$8
  Top 1.27: OUT3.1 10.13,33.81 Q3.3
N$10  (via drill 0.6)
  Top 0.406: R8.2 15.78,49.28 16.54,48.51 16.54,44.96 16.03,44.45 14.66,44.45 Q4.1 14.76,44.35 v14.76,42.93 | R7.2 86.2,8.32 81.82,11.68 73.44,11.68 64.04,11.68 v63.79,11.94
  Bottom 0.406: v63.79,11.94 29.5,11.94 19.59,21.84 19.59,38.1 v14.76,42.93
N$13  (via drill 0.6)
  Top 0.406: R6.2 15.53,39.37 16.54,38.35 16.54,35.56 16.03,35.05 14.66,35.05 Q3.1 14.51,35.03 v14.51,33.53 | R5.2 83.92,8.32 v81.06,10.67
  Bottom 0.406: v81.06,10.67 28.73,10.67 16.54,22.61 16.54,31.5 v14.51,33.53
N$14  (via drill 0.6)
  Top 0.406: R4.2 15.53,29.97 16.29,29.21 16.29,25.4 14.78,25.4 Q2.1 14.51,25.13 v14.51,23.11 | R3.2 81.31,8.38 80.04,9.65 v74.2,9.65
  Bottom 0.406: v74.2,9.65 27.21,9.65 v14.51,23.11
OUT1
  Top 0.406: B1.A11 79.28,5.4 R1.1
OUT2
  Top 0.406: B1.A12 81.82,5.4 R3.1
OUT3
  Top 0.406: B1.A13 84.36,5.4 R5.1
OUT4
  Top 0.406: B1.A14 86.9,5.4 R7.1
V_MOT
  Top 0.61: INT_PWR.2 23.4,4.57 25.69,6.86 25.69,30.23 22.89,33.02 22.89,37.34 23.91,38.35 25.69,38.35 PWR_FEEDER.2
  Top 1.016: PWR_FEEDER.2 31.78,38.61 C4.+ 32.43,37.96 C3.1 49.05,37.96 | 49.05,37.96 53.23,37.96 N0.2 N1.2 N2.2 N3.2 N4.2 N5.2 N6.2 N7.2 N8.2 N9.2 N10.2 N11.2 | 49.05,37.96 49.82,37.2 49.82,21.34 50.58,20.57 N12.2 N13.2 N14.2 N15.2 N16.2 N17.2 | N18.2 N19.2 N20.2 N21.2 N22.2 N23.2
  Bottom 1.016: N17.2 N18.2
V_PWR_OUTS
  Top 1.27: PWR_IN.2 11.74,8.1 C5.+ 14.76,8.13 14.76,8.38 12.48,10.67 2.06,10.67 1.3,11.43 1.3,16 3.56,18.26 OUT1.2 4.33,18.29 2.83,18.29 1.3,19.81 1.3,25.4 4.33,28.42 OUT2.2 1.3,31.47 1.3,36.32 3.82,38.84 OUT3.2 1.3,41.88 1.3,47.75 2.55,49 OUT4.2
VAC1  (via drill 0.6)
  Top 0.406: B1.A0 48.8,12.45 v46.77,14.48 | v41.43,14.73 38.89,14.73 VAC1.4
  Bottom 0.406: v46.77,14.48 41.69,14.48 v41.43,14.73
VAC2
  Top 0.406: VAC2.4 43.21,27.43 44.99,25.65 44.99,18.03 51.34,12.45 B1.A1

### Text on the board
tPlace: + | feedback | - | + | servo | + | feeder+ | feeder- | - | - | + | feedback | servo | - | feeder+ | + | feeder- | - | + | -
bPlace: 0816 feeder controller shield / up to 24 feeder / + 4 power-output / + 2 NXP vaccum sensors / / 2017/11/26 v2.2 / by mgrl / docs.mgrl.de / github.com/mgrl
